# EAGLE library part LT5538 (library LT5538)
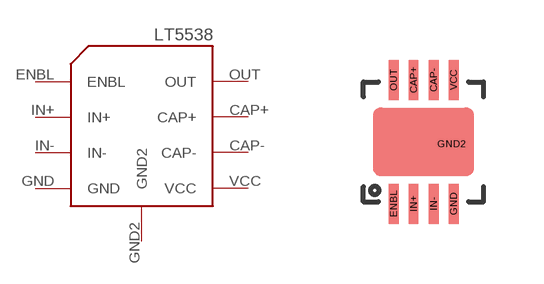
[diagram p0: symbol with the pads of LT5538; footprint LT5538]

Designator prefix -

## LT5538  [LT5538]
CAP+  CAP+
CAP-  CAP-
ENBL  ENBL
GND  GND  pwr
GND2  GND2
IN+  IN+
IN-  IN-
OUT  OUT  out
VCC  VCC  pwr

## Footprint LT5538 (pad centres in mm)
smd 0.25 x 1: CAP+ -0.22,1.58; CAP- 0.28,1.58; ENBL -0.72,-1.52; GND 0.78,-1.52; IN+ -0.22,-1.52; IN- 0.28,-1.52; OUT -0.72,1.58; VCC 0.78,1.58
smd 1 x 0.25: GND2 0.73,-0.02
